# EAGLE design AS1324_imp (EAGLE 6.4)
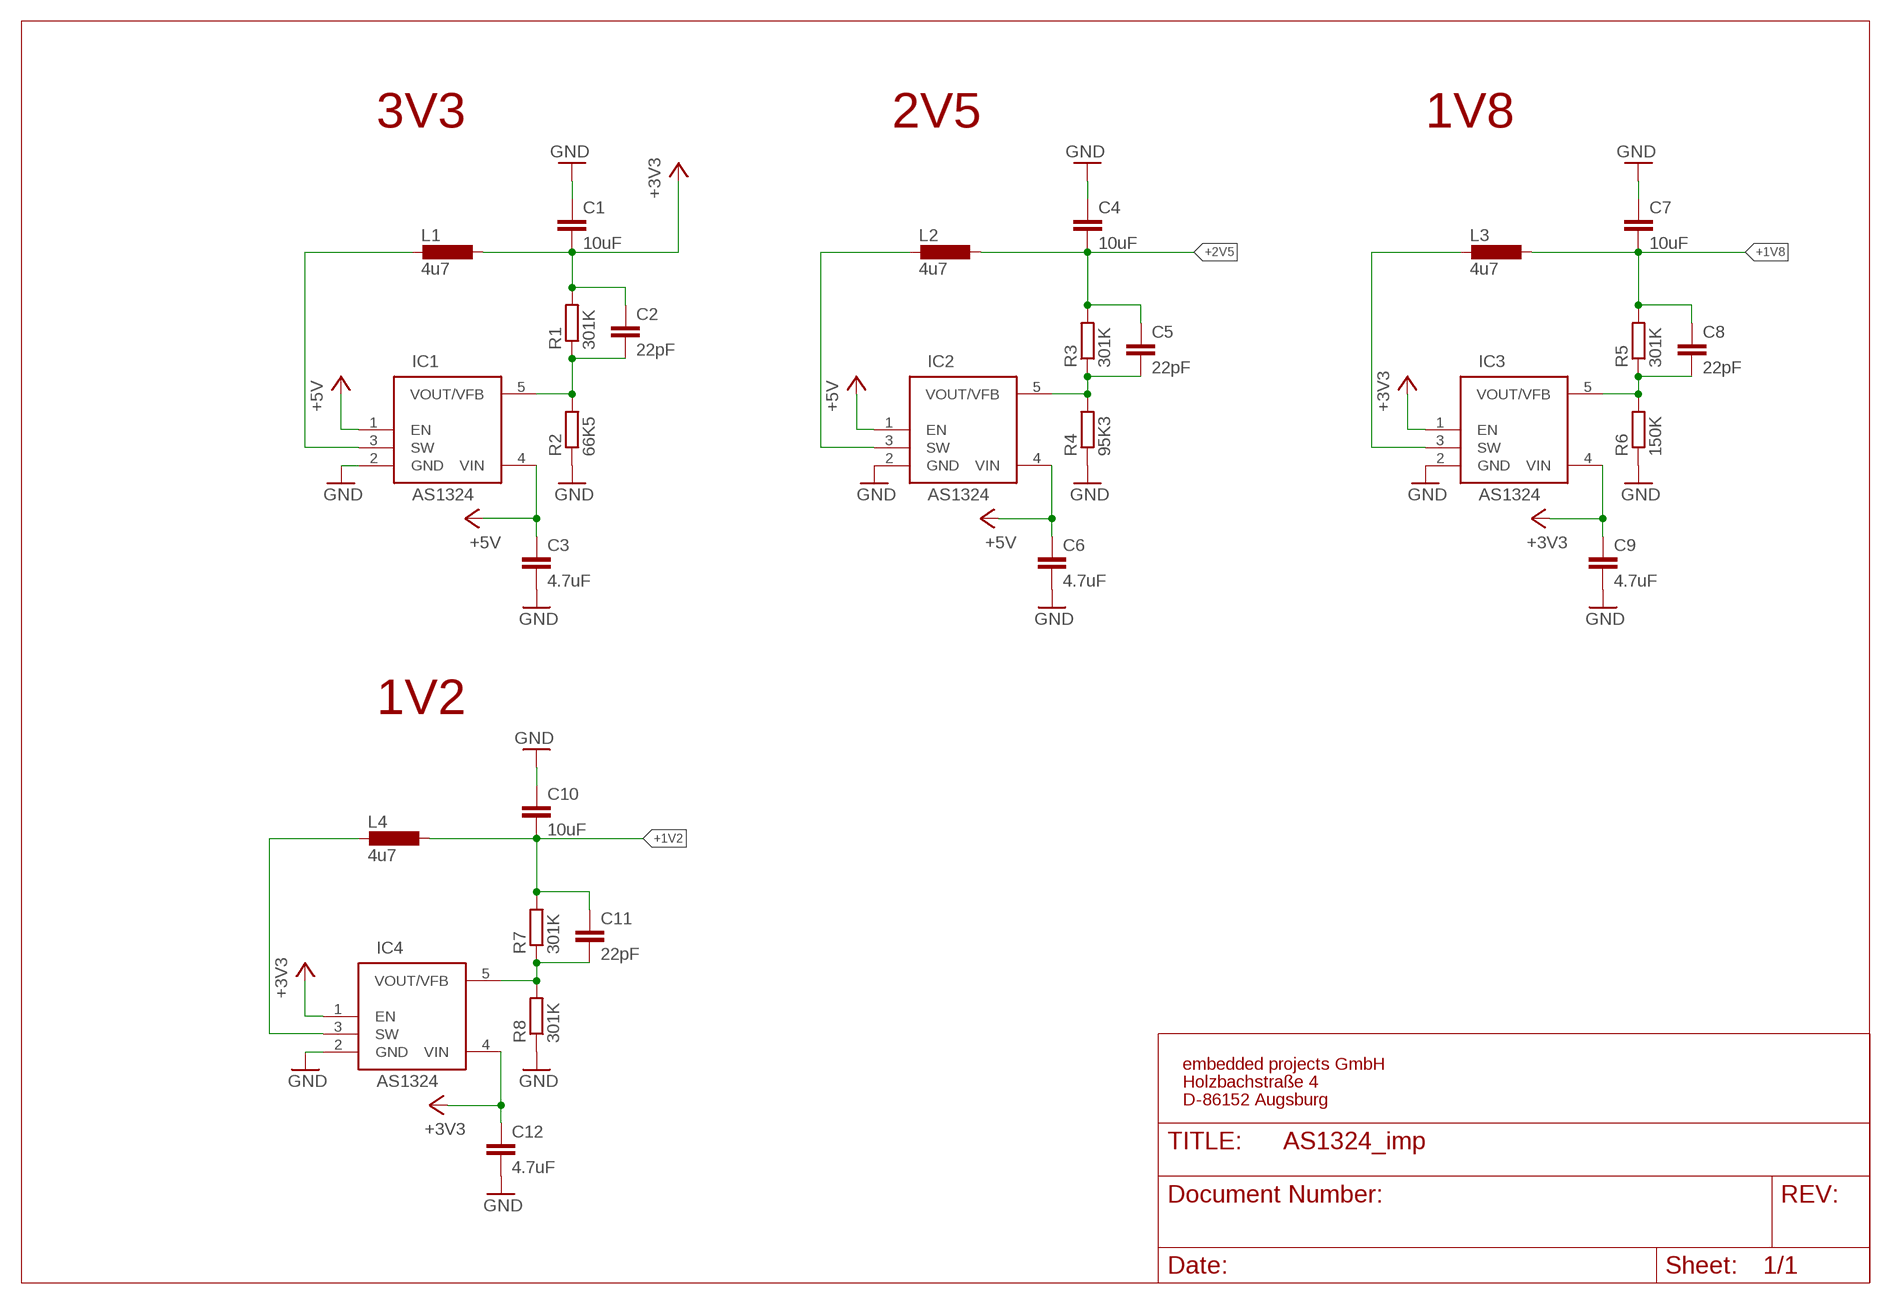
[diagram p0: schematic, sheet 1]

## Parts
C1  10uF  C-EUC0805  [C0805]
C2  22pF  C-EUC0805  [C0805]
C3  4.7uF  C-EUC0805  [C0805]
C4  10uF  C-EUC0805  [C0805]
C5  22pF  C-EUC0805  [C0805]
C6  4.7uF  C-EUC0805  [C0805]
C7  10uF  C-EUC0805  [C0805]
C8  22pF  C-EUC0805  [C0805]
C9  4.7uF  C-EUC0805  [C0805]
C10  10uF  C-EUC0805  [C0805]
C11  22pF  C-EUC0805  [C0805]
C12  4.7uF  C-EUC0805  [C0805]
IC1  AS1324  [TSOT23]
IC2  AS1324  [TSOT23]
IC3  AS1324  [TSOT23]
IC4  AS1324  [TSOT23]
L1  4u7  PSU3014  [PSU3014]
L2  4u7  PSU3014  [PSU3014]
L3  4u7  PSU3014  [PSU3014]
L4  4u7  PSU3014  [PSU3014]
R1  301K  R-EU_R0805  [R0805]
R2  66K5  R-EU_R0805  [R0805]
R3  301K  R-EU_R0805  [R0805]
R4  95K3  R-EU_R0805  [R0805]
R5  301K  R-EU_R0805  [R0805]
R6  150K  R-EU_R0805  [R0805]
R7  301K  R-EU_R0805  [R0805]
R8  301K  R-EU_R0805  [R0805]

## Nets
+1V2: C10.2 C11.1 L4.2 R7.2
+1V8: C7.2 C8.1 L3.2 R5.2
+2V5: C4.2 C5.1 L2.2 R3.2
+3V3: C1.2 C2.1 C9.1 C12.1 IC3.1(EN) IC3.4(VIN) IC4.1(EN) IC4.4(VIN) L1.2 R1.2
+5V: C3.1 C6.1 IC1.1(EN) IC1.4(VIN) IC2.1(EN) IC2.4(VIN)
GND: C1.1 C3.2 C4.1 C6.2 C7.1 C9.2 C10.1 C12.2 IC1.2(GND) IC2.2(GND) IC3.2(GND) IC4.2(GND) R2.1 R4.1 R6.1 R8.1
N$8: IC4.3(SW) L4.1
N$28: IC3.3(SW) L3.1
N$38: C11.2 IC4.5(VOUT/VFB) R7.1 R8.2
N$43: C8.2 IC3.5(VOUT/VFB) R5.1 R6.2
N$67: IC1.3(SW) L1.1
N$132: C2.2 IC1.5(VOUT/VFB) R1.1 R2.2
N$134: IC2.3(SW) L2.1
N$151: C5.2 IC2.5(VOUT/VFB) R3.1 R4.2

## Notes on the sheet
- 3V3 | 2V5 | 1V8
- 1V2
- embedded projects GmbH
- Holzbachstraße 4
- D-86152 Augsburg

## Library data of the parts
C1-C12 = rcl:C-EU: CAPACITOR, European symbol
IC1-IC4 = EmbeddedProjectsBauteile:AS1324: DC/DC Step-Down Regulator; EP: 400124
L1-L4 = KUBUS3B_PARTS2:PSU3014: SMD Power Inductors Shielded
R1-R8 = rcl:R-EU_: RESISTOR, European symbol

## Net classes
0 default: width 0.2 mm, drill 0.3 mm, clearance 0.2 mm
1 500mA: width 0.3 mm, drill 0.3 mm, clearance 0.15 mm
2 5V: width 0.305 mm, drill 0.4 mm, clearance 0.15 mm

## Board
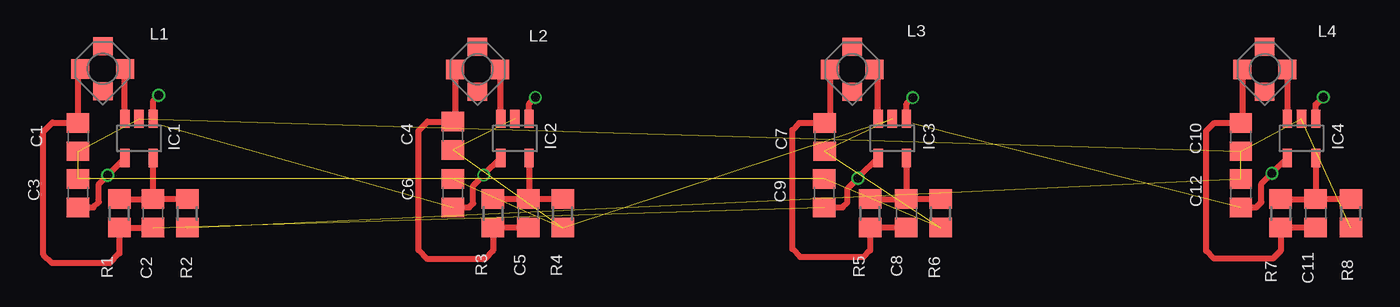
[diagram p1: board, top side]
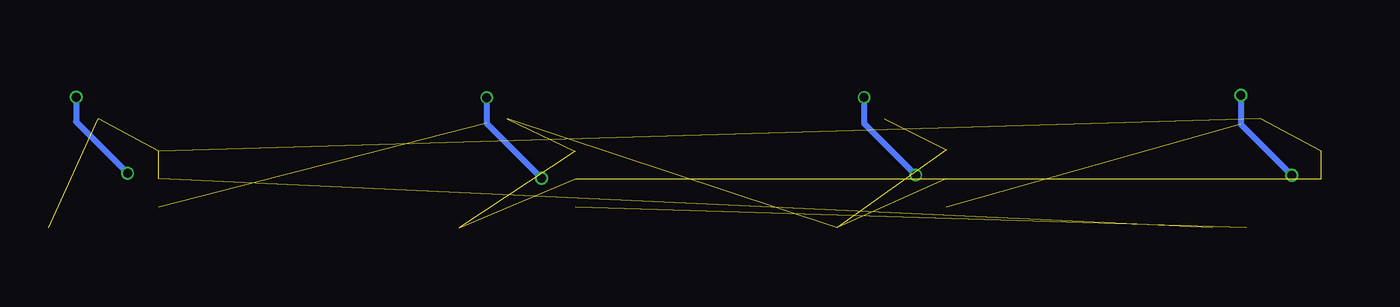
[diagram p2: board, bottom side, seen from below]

No outline drawn. Coordinates in mm, seen from the top.
Copper layers (1*2*15*16): Top 0.012mm / dielectric 0.36mm / Route2 0.018mm / dielectric 0.71mm / Route15 0.035mm / dielectric 0.2mm / Bottom 0.012mm
Design rules "125um_0.2mmborhung_4Layer *": minimum track width 0.125mm, minimum drill 0.25mm, track to track 0.125mm, track to pad 0.125mm, pad to pad 0.125mm, via to via 0.125mm, smd to smd 0mil, copper to edge 0.45mm, drill to drill 0.3mm, minimum pad ring 0.125mm, minimum via ring 0.125mm, stop-mask expansion 0.125mm, vias tented up to drill 40mil, thermal gap 0.2mm
bRestrict: area 51.6,54.2 to 59.1,60

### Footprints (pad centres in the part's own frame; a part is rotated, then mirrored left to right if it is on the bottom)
C0805 = smd 1.3 x 1.5: 1 -0.95,0; 2 0.95,0
TSOT23 = smd 0.622 x 1.22: 1 -0.95,-1.31; 2 0,-1.31; 3 0.95,-1.31; 4 0.95,1.31; 5 -0.95,1.31
PSU3014 = smd 1.2 x 1.3: 1 -1.5,0; 2 1.5,0 | smd 1.3 x 1.2: 3 0,1.5; 4 0,-1.5
R0805 = smd 1.3 x 1.5: 1 -0.95,0; 2 0.95,0

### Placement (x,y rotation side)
C1  11.71,32.23 90 top
C2  16.71,27.13 90 top
C3  11.7,28.48 90 top
C4  36.76,32.32 90 top
C5  41.81,27.13 90 top
C6  36.76,28.48 90 top
C7  61.62,32.23 90 top
C8  67.08,27.13 90 top
C9  61.58,28.48 90 top
C10  89.44,32.23 90 top
C11  94.45,27.13 90 top
C12  89.44,28.48 90 top
IC1  15.78,32.14 180 top
IC2  40.91,32.14 180 top
IC3  66.14,32.14 180 top
IC4  93.5,32.14 180 top
L1  13.36,36.79 180 top
L2  38.41,36.76 180 top
L3  63.46,36.76 180 top
L4  91.04,36.76 180 top
R1  14.47,27.13 270 top
R2  19.01,27.13 90 top
R3  39.44,27.13 270 top
R4  44.1,27.13 90 top
R5  64.66,27.13 270 top
R6  69.36,27.13 90 top
R7  92.1,27.13 270 top
R8  96.8,27.13 90 top

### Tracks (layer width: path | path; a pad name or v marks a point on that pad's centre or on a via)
+1V2
  Top 0.406: L4.2 89.54,33.28 C10.2 87.67,33.18 87.13,32.64 87.13,24.63 87.65,24.11 91.58,24.11 92.1,24.63 R7.2 C11.1
+1V8
  Top 0.406: L3.2 61.96,33.52 C7.2 59.92,33.17 59.45,32.7 59.45,24.75 59.99,24.21 64.21,24.21 64.66,24.66 R5.2 C8.1
+2V5
  Top 0.406: L2.2 36.91,33.42 C4.2 35.07,33.26 34.46,32.65 34.46,24.67 35.05,24.08 38.9,24.08 39.44,24.62 R3.2 C5.1
+3V3  (via drill 0.6)  (2 unrouted)
  Top 0.406: L1.2 11.71,36.64 C1.2 9.99,33.19 9.39,32.59 9.39,24.38 9.97,23.8 13.82,23.8 14.47,24.45 R1.2 C2.1 | IC3.1 67.09,34.45 v67.51,34.87 | IC3.4 63.96,29.6 v63.84,29.47 63.13,28.76 63.13,27.84 62.82,27.53 C9.1 | IC4.1 94.45,34.39 v94.96,34.9 | IC4.4 v91.52,29.8 v91.52,29.81 90.82,29.11 90.82,27.88 90.47,27.53 C12.1
  Bottom 0.406: v67.51,34.87 67.51,33.15 v63.84,29.47 | v94.96,34.9 94.97,33.26 v91.52,29.81
+5V  (via drill 0.6)  (1 unrouted)
  Top 0.406: IC1.1 16.73,34.66 v17.09,35.02 | IC1.4 v13.68,29.68 13.1,29.08 13.1,27.88 12.73,27.53 C3.1 | IC2.1 41.86,34.46 v42.28,34.88 | IC2.4 v38.83,29.7 v38.83,29.69 38.12,28.98 38.12,27.8 37.85,27.53 C6.1
  Bottom 0.406: v17.09,35.02 17.09,33.09 v13.68,29.68 | v42.28,34.88 42.28,33.14 v38.83,29.69
GND  (15 unrouted)
N$8
  Top 0.406: L4.1 IC4.3
N$28
  Top 0.406: IC3.3 65.19,36.53 L3.1
N$38
  Top 0.406: R7.1 C11.2 | R8.2 C11.2 | IC4.5 C11.2
N$43
  Top 0.406: R6.2 C8.2 | R5.1 C8.2 | IC3.5 C8.2
N$67
  Top 0.406: IC1.3 14.83,36.76 L1.1
N$132
  Top 0.406: R1.1 C2.2 | R2.2 C2.2 | C2.2 16.71,30.81 IC1.5
N$134
  Top 0.406: IC2.3 39.96,36.71 L2.1
N$151
  Top 0.406: IC2.5 41.86,28.13 C5.2 | R4.2 C5.2 | C5.2 R3.1

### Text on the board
Document: 5V auf 3,3V | 5V auf 2,5V | 3,3V auf 1,8V | 3,3V auf 1,2V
